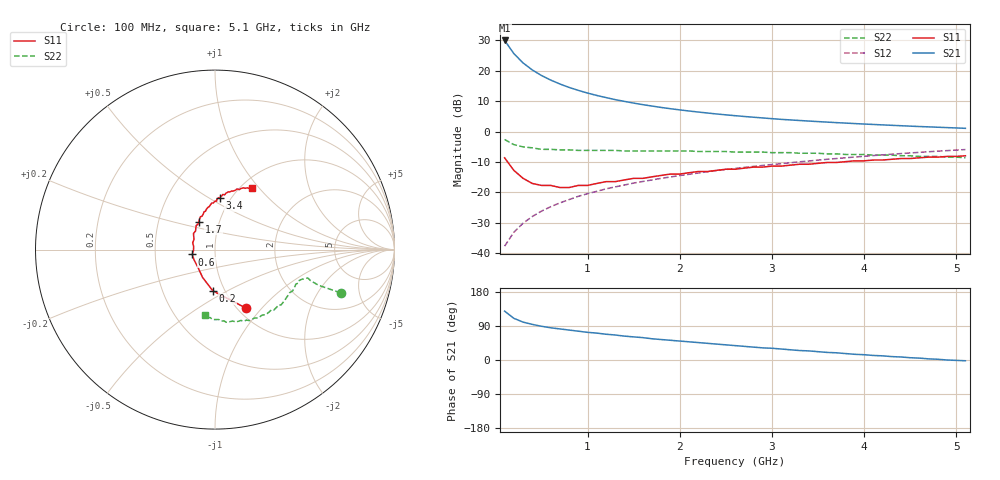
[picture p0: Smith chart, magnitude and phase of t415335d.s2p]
!AT-41533
!S and NOISE PARAMETERS at Vce=5V Ic=25mA. LAST UPDATED 01-25-95
# ghz s ma r 50
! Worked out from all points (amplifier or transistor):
!   51 points, 100 MHz to 5.1 GHz, reference 50 ohm
!   highest |S21| = 30.0 dB at 100 MHz (marker M1)
!   |S21| within 3 dB of that: start of sweep to 169.7 MHz
!   unconditionally stable (mu >= 1): 423.6 MHz to 2.052 GHz
!   at 900 MHz: K = 1.05, MAG = 16.0 dB, |S12| = -21.3 dB
!   at 2.6 GHz: K = 0.97, MSG = 8.7 dB, |S12| = -12.1 dB
!   at 5.1 GHz: K = 0.87, MSG = 3.5 dB, |S12| = -5.9 dB
!   lowest NFmin = 1.30 dB at 100 MHz
!   S11 on the Smith chart (normalised r, x): 100 MHz: 1.09, -0.83; 200 MHz: 0.88, -0.43; 600 MHz: 0.77, -0.04; 1.7 GHz: 0.80, +0.26; 3.4 GHz: 0.89, +0.56; 5.1 GHz: 1.12, +0.92
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0.1  0.37 -62.0  31.61 129.0  0.013 73.0  0.74 -19.0
0.2  0.23 -93.0  19.25 110.0  0.022 73.0  0.61 -19.0
0.3  0.17 -114.0  13.49 100.0  0.031 75.0  0.56 -18.0
0.4  0.14 -131.0  10.34 94.0  0.04 76.0  0.54 -17.0
0.5  0.13 -153.0  8.375 89.0  0.049 76.0  0.51 -19.0
0.6  0.13 -168.0  7.042 85.0  0.058 76.0  0.51 -19.0
0.7  0.12 -177.0  6.07 82.0  0.067 76.0  0.5 -20.0
0.8  0.12 172.0  5.329 79.0  0.076 76.0  0.5 -22.0
0.9  0.13 163.0  4.764 76.0  0.086 75.0  0.49 -23.0
1  0.13 154.0  4.305 73.0  0.095 74.0  0.49 -25.0
1.2  0.15 143.0  3.629 68.0  0.114 73.0  0.49 -27.0
1.3  0.15 136.0  3.357 66.0  0.123 72.0  0.49 -28.0
1.4  0.16 132.0  3.139 63.0  0.132 71.0  0.48 -30.0
1.7  0.18 120.0  2.63 56.0  0.16 69.0  0.48 -34.0
1.8  0.19 117.0  2.493 54.0  0.17 68.0  0.48 -35.0
2.2  0.22 106.0  2.098 46.0  0.208 64.0  0.47 -41.0
2.6  0.24 98.0  1.827 38.0  0.247 60.0  0.46 -47.0
2.9  0.26 92.0  1.677 32.0  0.277 57.0  0.46 -52.0
3.4  0.29 85.0  1.49 24.0  0.328 52.0  0.44 -62.0
3.5  0.3 83.0  1.46 22.0  0.339 51.0  0.44 -64.0
4.3  0.35 71.0  1.268 9.0  0.424 41.0  0.41 -81.0
5.1  0.4 59.0  1.131 -2.0  0.506 31.0  0.37 -99.0
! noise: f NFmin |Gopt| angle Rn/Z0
0.1  1.3  0.08  13  0.12
0.9  1.6  0.19  -170  0.1
1.8  1.9  0.42  -126  0.16
2.4  2.1  0.55  -105  0.32
